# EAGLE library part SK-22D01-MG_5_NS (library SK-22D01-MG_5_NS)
Slide Switches DPDT 0.3 Amp at 30 V Source: Datasheet
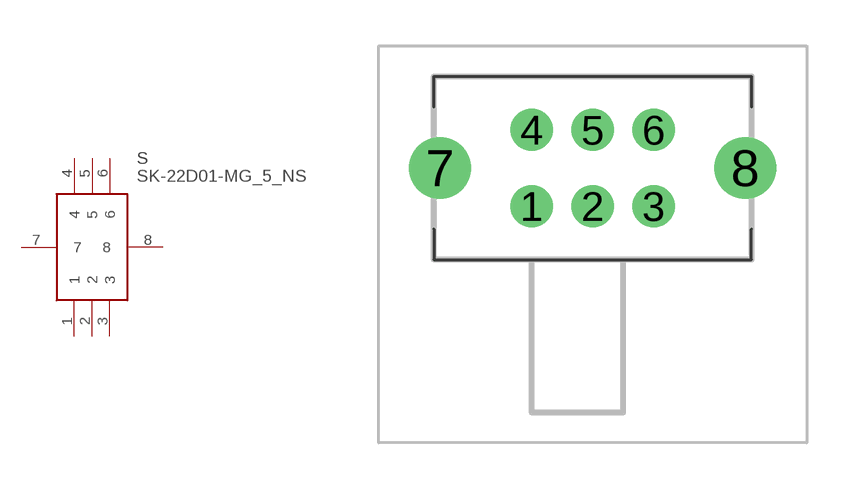
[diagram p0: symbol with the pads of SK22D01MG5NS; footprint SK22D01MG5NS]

Designator prefix S

## SK-22D01-MG_5_NS (Arrow_Part_Number: SK-22D01-MG 5 NS; Arrow_Price-Stock: https://www.arrow.com/en/products/sk22d01mg5ns/ck?region=nac; Description: Slide Switches DPDT 0.3 Amp at 30 V; Height: 5.1mm; Manufacturer_Name: C & K COMPONENTS; Manufacturer_Part_Number: SK-22D01-MG 5 NS; Mouser_Part_Number: 611-SK-22D01-MG5NS; Mouser_Price-Stock: https://www.mouser.co.uk/ProductDetail/CK/SK-22D01-MG-5-NS?qs=T%252BgPUmif8%252Bj%2Ffo3NJcSFGw%3D%3D)  [SK22D01MG5NS]
1  1
2  2
3  3
4  4
5  5
6  6
7  7
8  8

## Footprint SK22D01MG5NS (pad centres in mm)
SK-22D01-MG 5 NS-2
drill 0.85 pad 1.381: 1 0,0; 2 2,0; 3 4,0; 4 0,2.5; 5 2,2.5; 6 4,2.5
drill 1.35 pad 2.025: 7 -3,1.25; 8 7,1.25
